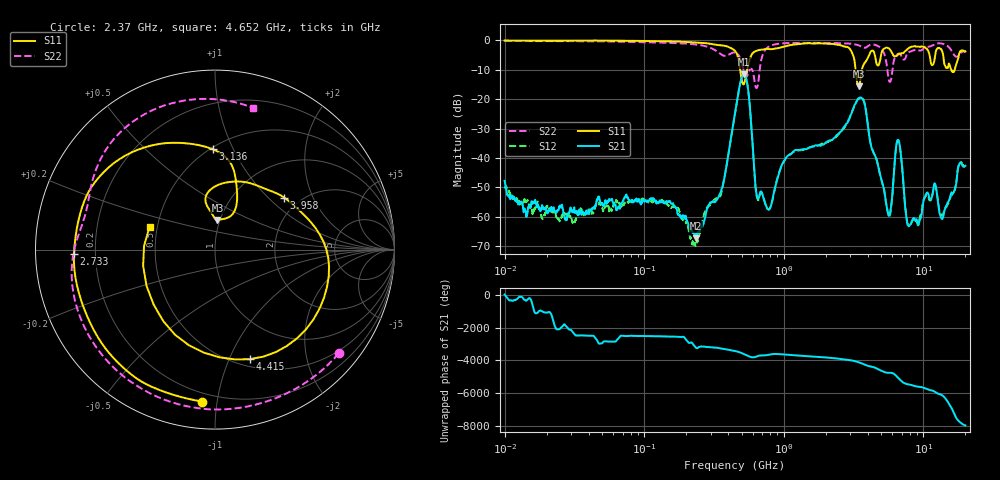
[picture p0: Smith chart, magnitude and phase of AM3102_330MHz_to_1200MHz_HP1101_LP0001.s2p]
! Date/Time: Tue, Sep 11, 2018 5:21 PM
! Network Analyzer: Agilent Technologies E8362B Rev: A.07.50.63
! Sweep from 0.010 to 20.000 GHz, 1601 Points, Sweep Type: LOG
! Power Supply: 4.949 V, 0.001 A
# Hz S DB R 50
!freq MagS11 AngS11 MagS21 AngS21 MagS12 AngS12 MagS22 AngS22
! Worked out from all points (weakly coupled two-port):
!   1601 points, 10 MHz to 20 GHz, reference 50 ohm
!   highest |S21| = -11.51 dB at 518.2 MHz (marker M1); lowest = -67.3 dB at 234.4 MHz (marker M2)
!   lowest |S11| = -15.6 dB at 3.449 GHz (marker M3), VSWR 1.40, Z = 48.6 + j16.5 ohm
!   |S11| at or under -10 dB: 486.3 MHz to 547.1 MHz (60.79 MHz wide, 11.8 % of centre); 3.267 GHz to 3.626 GHz (358.9 MHz wide, 10.4 % of centre); 15.86 GHz to 16.75 GHz (885.1 MHz wide, 5.43 % of centre)
!   |S22| runs from -16.2 to -0.2 dB; largest |S21 - S12| = 0.0056
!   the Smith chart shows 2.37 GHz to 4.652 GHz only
!   S11 on the Smith chart (normalised r, x): 2.37 GHz: 0.15, -0.91; 2.733 GHz: 0.12, -0.02; 3.136 GHz: 0.51, +0.84; 3.958 GHz: 1.66, +1.26; 4.415 GHz: 0.58, -1.19; 4.652 GHz: 0.45, +0.13
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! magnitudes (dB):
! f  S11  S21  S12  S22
! 10 MHz  0.0  -47.8  -50.4  -0.2
! 35.55 MHz  -0.1  -59.4  -57.4  -0.3
! 126.4 MHz  -0.2  -55.5  -54.9  -0.7
! 234.4 MHz  -0.7  -67.3  -69.8  -1.4
! 356 MHz  -1.7  -51.1  -52.2  -4.8
! 447.2 MHz  -3.6  -24.8  -24.8  -4.1
! 518.2 MHz  -14.8  -11.5  -11.5  -10.7
! 641.7 MHz  -3.5  -53.0  -53.3  -16.1
! 765 MHz  -2.9  -57.3  -57.3  -2.4
! 1.59 GHz  -1.0  -36.2  -36.1  -0.8
! 2.37 GHz  -1.4  -32.4  -32.8  -0.9
! 2.733 GHz  -2.1  -29.1  -29.5  -1.0
! 3.136 GHz  -5.0  -23.4  -23.4  -1.2
! 3.449 GHz  -15.6  -19.7  -19.7  -1.7
! 3.958 GHz  -6.3  -27.1  -27.0  -2.1
! 4.415 GHz  -3.9  -38.4  -38.3  -1.4
! 4.652 GHz  -8.3  -41.0  -41.1  -1.7
! 5.652 GHz  -2.7  -59.6  -60.0  -13.5
! 6.58 GHz  -4.7  -33.8  -34.0  -4.6
! 7.92 GHz  -2.5  -63.2  -62.9  -3.9
! 13.68 GHz  -3.9  -60.8  -59.5  -1.1
! 20 GHz  -3.8  -42.7  -43.2  -3.8
